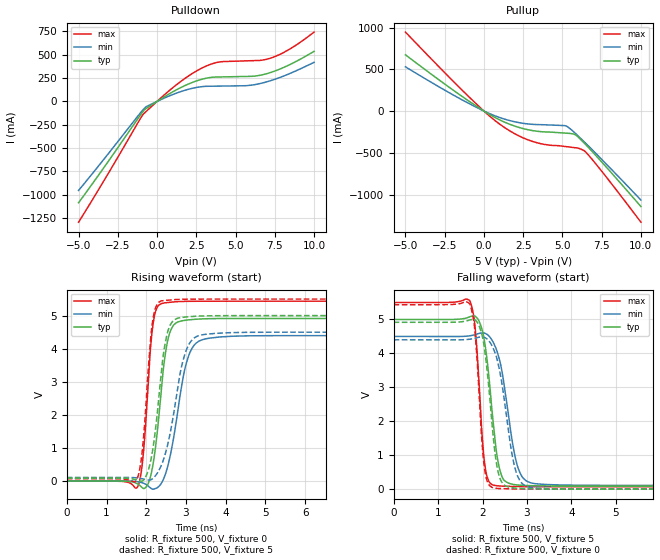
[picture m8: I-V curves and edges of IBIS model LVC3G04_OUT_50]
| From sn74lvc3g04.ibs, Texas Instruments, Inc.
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[Model]   LVC3G04_OUT_50
Model_type  Output
Vref =   0
Rref =   500
Cref =   50p
Vmeas =   2.5
| variable   typ   min   max
C_comp   8.92pF   5.46pF   12.38pF
| C_pullup   9.70pF   5.46pF   12.38pF
| C_pulldown   8.14pF   6.08pF   10.97pF
[Temperature Range]   40   100   -40
| Ambient temperature   25   85   -40
[Voltage range]   5   4.5   5.5
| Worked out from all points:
|   slope of the pulldown table from 0 to 0.75 V, typ, clamps not added: 9.57 ohm
|   slope of the pullup table from 0 to 0.75 V, typ, clamps not added: 9.17 ohm
|   rising waveform, R_fixture 500, V_fixture 0: 20-80 % time 264ps typ, 377ps min, 187ps max; typ from 0 V to 4.91 V
|   falling waveform, R_fixture 500, V_fixture 5: 20-80 % time 234ps typ, 312ps min, 160ps max; typ from 5 V to 0.09 V
|   rising waveform, R_fixture 500, V_fixture 5: 20-80 % time 277ps typ, 406ps min, 199ps max; typ from 0.09 V to 5 V
|   falling waveform, R_fixture 500, V_fixture 0: 20-80 % time 224ps typ, 305ps min, 158ps max; typ from 4.92 V to 0 V
[Pulldown]
| LVC3G04_OUT_50
|   Voltage   I(typ)   I(min)   I(max)
-5V       -1.085A    -953mA     -1.293A
-925mV    -115.1mA   -95.62mA   -147.4mA
-625mV    -68.8mA    -50.72mA   -96.83mA
1.06V     108.1mA    77.61mA    154.7mA
2.425V    214.3mA    146.7mA    317.2mA
3.59V     259.5mA    163mA      407.1mA
4.175V    262.2mA    164.4mA    426.1mA
5.89V     268.1mA    171.9mA    435.3mA
6.74V     286.3mA    198.6mA    443mA
7.465V    323mA      234.9mA    477.5mA
8.625V    408mA      310.8mA    578.1mA
10V       536.4mA    418mA      742.1mA
[Pullup]
| LVC3G04_OUT_50
|   Voltage   I(typ)   I(min)   I(max)
-5V       673.9mA    530.1mA    946.1mA
-985mV    122.4mA    93.65mA    175.9mA
240mV     -27.95mA   -20.84mA   -40.82mA
1.115V    -115.9mA   -84.71mA   -171.7mA
2.1V      -188.7mA   -134mA     -285.4mA
3.08V     -233.7mA   -159.1mA   -363.2mA
3.96V     -250.6mA   -165.4mA   -403mA
5.285V    -265.7mA   -183.8mA   -427.4mA
5.82V     -284mA     -266.4mA   -439.7mA
6.485V    -402.3mA   -386.4mA   -491.6mA
7.725V    -656.8mA   -621.8mA   -774mA
10V       -1.144A    -1.066A    -1.332A
[Ramp]
| LVC3G04_OUT_50
| variable   typ   min   max
dV/dt_r   3.08/2.84E-10   2.78/4.07E-10   3.39/2.00E-10
dV/dt_f   3.01/2.51E-10   2.70/3.24E-10   3.32/1.72E-10
R_load = 500
[Rising Waveform]
| LVC3G04_OUT_50
R_fixture =   500
C_fixture =   0
L_fixture =   0
V_fixture =   0
V_fixture_min = 0
V_fixture_max = 0
|   Time   V(typ)   V(min)   V(max)
0s        181.8pV    4.332nV    2.343nV
1.79ns    -89.87mV   -20.33mV   -156.7mV
1.93ns    -226.4mV   -63.32mV   870.2mV
2.095ns   83.14mV    -197.1mV   3.822V
2.165ns   466.2mV    -243.2mV   4.686V
2.4ns     3.006V     -25.57mV   5.371V
2.615ns   4.554V     833mV      5.404V
3.05ns    4.868V     3.724V     5.431V
3.585ns   4.907V     4.318V     5.435V
24.99ns   4.914V     4.397V     5.435V
[Falling Waveform]
| LVC3G04_OUT_50
R_fixture =   500
C_fixture =   0
L_fixture =   0
V_fixture =   5
V_fixture_min = 4.5
V_fixture_max = 5.5
|   Time   V(typ)   V(min)   V(max)
0s        5V         4.5V       5.5V
1.715ns   5.081V     4.52V      5.55V
1.84ns    5.09V      4.555V     4.672V
2.05ns    4.312V     4.595V     739.8mV
2.14ns    3.364V     4.518V     237.9mV
2.285ns   1.416V     4.206V     106.2mV
2.455ns   319.8mV    3.338V     89.14mV
2.78ns    124.3mV    711.2mV    76.98mV
3.185ns   99.87mV    161mV      72.06mV
24.99ns   89.64mV    109.7mV    70.16mV
[Rising Waveform]
| LVC3G04_OUT_50
R_fixture =   500
C_fixture =   0
L_fixture =   0
V_fixture =   5
V_fixture_min = 4.5
V_fixture_max = 5.5
|   Time   V(typ)   V(min)   V(max)
0s        89.62mV    109.7mV    70.15mV
1.75ns    40.57mV    98.19mV    21.77mV
1.905ns   7.764mV    68.73mV    974.2mV
2.1ns     543.8mV    36.59mV    4.134V
2.215ns   1.391V     138mV      5.162V
2.39ns    3.389V     506.2mV    5.448V
2.595ns   4.694V     1.408V     5.471V
2.98ns    4.956V     3.86V      5.495V
3.475ns   4.992V     4.433V     5.499V
24.99ns   5V         4.5V       5.5V
[Falling Waveform]
| LVC3G04_OUT_50
R_fixture =   500
C_fixture =   0
L_fixture =   0
V_fixture =   0
V_fixture_min = 0
V_fixture_max = 0
|   Time   V(typ)   V(min)   V(max)
0s        4.917V     4.401V     5.437V
1.715ns   4.988V     4.419V     5.452V
1.835ns   4.985V     4.449V     4.564V
1.975ns   4.607V     4.485V     1.632V
2.045ns   4.137V     4.471V     612.2mV
2.29ns    975.1mV    3.99V      26.95mV
2.43ns    214.2mV    3.164V     16.08mV
2.735ns   31.6mV     602.5mV    6.711mV
3.095ns   9.906mV    46.77mV    2.166mV
24.99ns   19.27uV    21.35uV    15.34uV
